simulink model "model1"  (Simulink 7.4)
settings: Solver=ode4  StartTime=0.0  StopTime=1  FixedStep=1e-4  RelTol=1e-3
libraries: simulink x2

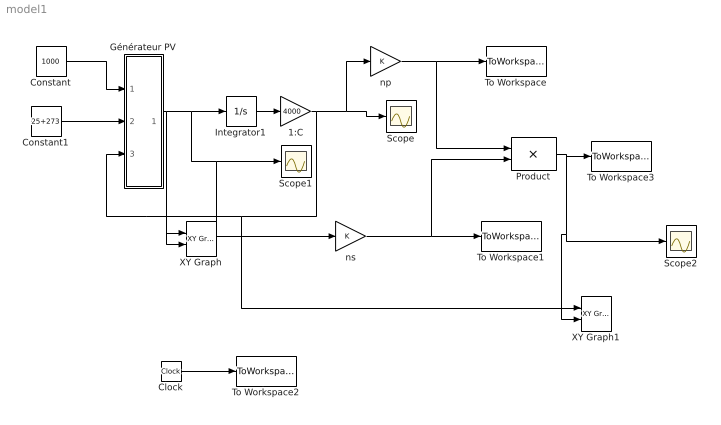
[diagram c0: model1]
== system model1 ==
  1:C : Gain  Gain=4000  ParameterDataType=sfix(16)  ParameterScaling=2^0  OutDataType=sfix(16)  OutScaling=2^0
  Clock : Clock
  Constant : Constant  Value=1000  OutDataType=sfix(16)  OutScaling=2^0
  Constant1 : Constant  Value=25+273  OutDataType=sfix(16)  OutScaling=2^0
  Générateur PV : Subsystem
  Integrator1 : Integrator
  Product : Product  OutDataType=sfix(16)  OutScaling=2^0
  Scope : Scope
  Scope1 : Scope
  Scope2 : Scope
  To Workspace : ToWorkspace  VariableName=Vpv  SampleTime=-1  SaveFormat=Array
  To Workspace1 : ToWorkspace  VariableName=Ipv  SampleTime=-1  SaveFormat=Array
  To Workspace2 : ToWorkspace  VariableName=t  SampleTime=-1  SaveFormat=Array
  To Workspace3 : ToWorkspace  VariableName=Ppv  SampleTime=-1  SaveFormat=Array
  XY Graph : simulink/Sinks/XY Graph  SystemSampleTime=-1  xmin=0  xmax=50  ymin=01  ymax=5  st=-1
  XY Graph1 : simulink/Sinks/XY Graph  SystemSampleTime=-1  xmin=0  xmax=50  ymin=01  ymax=120  st=-1
  np : Gain  ParameterDataType=sfix(16)  ParameterScaling=2^0  OutDataType=sfix(16)  OutScaling=2^0
  ns : Gain  ParameterDataType=sfix(16)  ParameterScaling=2^0  OutDataType=sfix(16)  OutScaling=2^0
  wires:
  Integrator1/1 -> 1:C/1
  1:C/1 -> Scope/1, np/1, Générateur PV/3(VG), XY Graph/1, XY Graph1/1
  Générateur PV/1(IG) -> Integrator1/1, Scope1/1, ns/1, XY Graph/2
  Constant/1 -> Générateur PV/1(Es)
  Clock/1 -> To Workspace2/1
  Constant1/1 -> Générateur PV/2(Tj)
  ns/1 -> To Workspace1/1, Product/2
  Product/1 -> To Workspace3/1, Scope2/1, XY Graph1/2
  np/1 -> Product/1, To Workspace/1

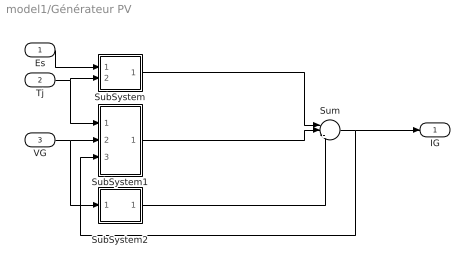
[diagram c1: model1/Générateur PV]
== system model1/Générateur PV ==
  Es : Inport  OutDataType=sfix(16)  OutScaling=2^0
  Tj : Inport  Port=2  OutDataType=sfix(16)  OutScaling=2^0
  VG : Inport  Port=3  OutDataType=sfix(16)  OutScaling=2^0
  SubSystem : Subsystem  mask{Tjref=298, Eref=1000, p3=-0.336e-4, p2=0.58e-5, p1=0.00345}
      mask prompts: Tjref "Tjref[°k]"; Eref "Eref[W/m^2]"
  SubSystem1 : Subsystem  mask{Rs=0.92251, ns=72, p4=31.2367, Eg=1.76e-19, q=1.6e-19, A=1, k=1.38e-23}
      mask prompts: Rs "Rs[ohm]"; q "q[C]"; k "k[J/°K]"
  SubSystem2 : Subsystem  mask{Rsh=235.1551}
      mask prompts: Rsh "Rsh[ohm]"
  Sum : Sum  Inputs=|+--  OutDataType=sfix(16)  OutScaling=2^0
  IG : Outport  OutDataType=sfix(16)  OutScaling=2^0
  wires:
  SubSystem/1(Iph) -> Sum/1
  SubSystem1/1(Id) -> Sum/2
  SubSystem2/1(Irsh) -> Sum/3
  Es/1 -> SubSystem/1(Es)
  Tj/1 -> SubSystem/2(Tj), SubSystem1/1(Tj)
  Sum/1 -> IG/1, SubSystem1/3(IG)
  VG/1 -> SubSystem1/2(VG), SubSystem2/1(VG)

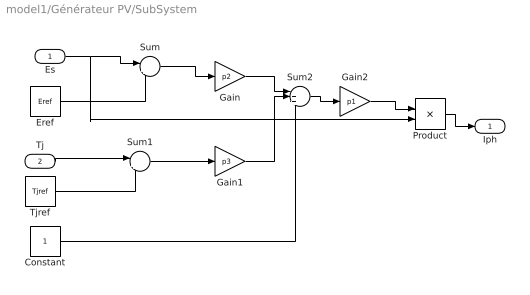
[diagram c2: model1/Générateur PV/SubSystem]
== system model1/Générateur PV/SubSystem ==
  Es : Inport  OutDataType=sfix(16)  OutScaling=2^0
  Tj : Inport  Port=2  OutDataType=sfix(16)  OutScaling=2^0
  Constant : Constant  OutDataType=sfix(16)  OutScaling=2^0
  Eref : Constant  Value=Eref  OutDataType=sfix(16)  OutScaling=2^0
  Gain : Gain  Gain=p2  ParameterDataType=sfix(16)  ParameterScaling=2^0  OutDataType=sfix(16)  OutScaling=2^0
  Gain1 : Gain  Gain=p3  ParameterDataType=sfix(16)  ParameterScaling=2^0  OutDataType=sfix(16)  OutScaling=2^0
  Gain2 : Gain  Gain=p1  ParameterDataType=sfix(16)  ParameterScaling=2^0  OutDataType=sfix(16)  OutScaling=2^0
  Product : Product  OutDataType=sfix(16)  OutScaling=2^0
  Sum : Sum  Inputs=|+-  OutDataType=sfix(16)  OutScaling=2^0
  Sum1 : Sum  Inputs=|+-  OutDataType=sfix(16)  OutScaling=2^0
  Sum2 : Sum  Inputs=|+++  OutDataType=sfix(16)  OutScaling=2^0
  Tjref : Constant  Value=Tjref  OutDataType=sfix(16)  OutScaling=2^0
  Iph : Outport  OutDataType=sfix(16)  OutScaling=2^0
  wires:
  Eref/1 -> Sum/2
  Tj/1 -> Sum1/1
  Tjref/1 -> Sum1/2
  Sum/1 -> Gain/1
  Sum1/1 -> Gain1/1
  Gain/1 -> Sum2/1
  Gain1/1 -> Sum2/2
  Constant/1 -> Sum2/3
  Sum2/1 -> Gain2/1
  Gain2/1 -> Product/1
  Es/1 -> Sum/1, Product/2
  Product/1 -> Iph/1

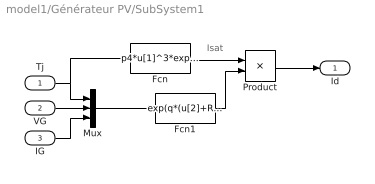
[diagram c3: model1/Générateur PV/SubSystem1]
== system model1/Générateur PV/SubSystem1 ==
  note: Isat
  Tj : Inport  OutDataType=sfix(16)  OutScaling=2^0
  VG : Inport  Port=2  OutDataType=sfix(16)  OutScaling=2^0
  IG : Inport  Port=3  OutDataType=sfix(16)  OutScaling=2^0
  Fcn : Fcn  Expr=p4*u[1]^3*exp(-Eg/(k*u[1]))
  Fcn1 : Fcn  Expr=exp(q*(u[2]+Rs*u[3])/(k*A*ns*u[1]))-1
  Mux : Mux  Inputs=3
  Product : Product  OutDataType=sfix(16)  OutScaling=2^0
  Id : Outport  OutDataType=sfix(16)  OutScaling=2^0
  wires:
  Mux/1 -> Fcn1/1
  Fcn/1 -> Product/1
  Fcn1/1 -> Product/2
  Product/1 -> Id/1
  VG/1 -> Mux/2
  IG/1 -> Mux/3
  Tj/1 -> Mux/1, Fcn/1

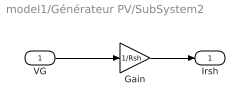
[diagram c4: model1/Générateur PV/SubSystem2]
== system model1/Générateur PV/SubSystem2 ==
  VG : Inport  OutDataType=sfix(16)  OutScaling=2^0
  Gain : Gain  Gain=1/Rsh  ParameterDataType=sfix(16)  ParameterScaling=2^0  OutDataType=sfix(16)  OutScaling=2^0
  Irsh : Outport  OutDataType=sfix(16)  OutScaling=2^0
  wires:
  VG/1 -> Gain/1
  Gain/1 -> Irsh/1
